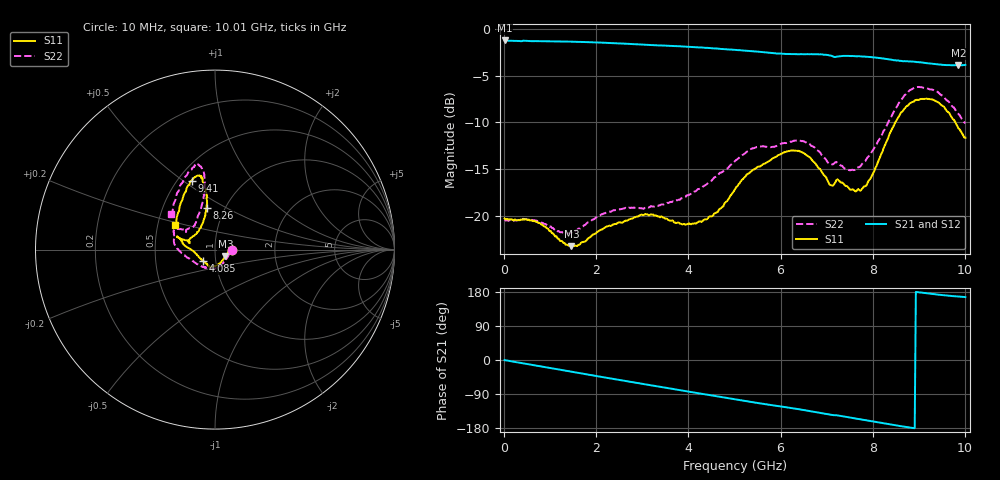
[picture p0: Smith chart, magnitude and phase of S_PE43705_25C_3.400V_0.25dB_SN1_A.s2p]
! Device ID: PE43705
! Serial: 1
! Insertion: A
! Impedance: 50 ohm
! Temp: 25C
! VDD: 3.400V
! Attenuation Step: 0.25dB
#  Hz  S  RI  R  50
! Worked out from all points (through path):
!   401 points, 10 MHz to 10.01 GHz, reference 50 ohm
!   highest |S21| = -1.26 dB at 10 MHz (marker M1); lowest = -3.9 dB at 9.86 GHz (marker M2)
!   group delay of S21, straight-line fit = 55.1 ps
!   lowest |S11| = -23.2 dB at 1.46 GHz (marker M3), VSWR 1.15, Z = 56 - j4.22 ohm
!   |S11| at or under -10 dB: start of sweep to 8.487 GHz; 9.793 GHz to end of sweep
!   |S22| runs from -21.9 to -6.2 dB; largest |S21 - S12| = 0.007
!   S11 on the Smith chart (normalised r, x): 10 MHz: 1.22, -0.00; 4.085 GHz: 0.87, -0.11; 8.26 GHz: 0.82, +0.41; 9.41 GHz: 0.59, +0.54; 10.01 GHz: 0.61, +0.18
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1e7  0.0973 -0.000861  0.8647 -0.0043  0.8654 -0.0041  0.0962 -0.00072
7.1e8  0.0926 0.0127  0.8281 -0.2221  0.8283 -0.2219  0.0945 0.00635
1.46e9  0.0582 -0.0375  0.7313 -0.4365  0.7316 -0.4366  0.0629 -0.0519
1.685e9  0.044 -0.0578  0.6905 -0.4943  0.6905 -0.4944  0.0465 -0.0742
2.235e9  0.00934 -0.0879  0.5704 -0.6155  0.5709 -0.6151  0.00145 -0.1052
3.36e9  -0.0321 -0.0943  0.2749 -0.7658  0.2758 -0.7653  -0.0576 -0.0987
4.085e9  -0.0646 -0.0646  0.0693 -0.7943  0.0698 -0.7942  -0.1131 -0.0723
4.585e9  -0.0986 -0.0321  -0.0717 -0.7811  -0.0709 -0.7807  -0.1557 -0.0444
5.01e9  -0.1392 0.00396  -0.1835 -0.7478  -0.1832 -0.7479  -0.1965 -0.00846
5.41e9  -0.1749 0.0278  -0.2795 -0.7027  -0.2789 -0.7035  -0.2277 0.0356
6.085e9  -0.2078 0.0713  -0.4115 -0.6074  -0.4086 -0.6065  -0.2288 0.0903
6.685e9  -0.1896 0.0594  -0.5227 -0.5099  -0.523 -0.509  -0.2059 0.1162
7.085e9  -0.14 0.0433  -0.5834 -0.4193  -0.5844 -0.4201  -0.1622 0.099
7.26e9  -0.1458 0.0536  -0.5948 -0.3908  -0.5929 -0.3921  -0.1501 0.1162
7.685e9  -0.1001 0.0974  -0.6491 -0.2955  -0.6482 -0.2954  -0.1108 0.145
7.91e9  -0.0754 0.1349  -0.6645 -0.2375  -0.6654 -0.2413  -0.0959 0.1853
8.26e9  -0.0469 0.2336  -0.6744 -0.1501  -0.6717 -0.1553  -0.0645 0.2829
8.36e9  -0.0448 0.2691  -0.6742 -0.1257  -0.6727 -0.1288  -0.0595 0.3208
8.86e9  -0.077 0.3993  -0.6672 -0.00925  -0.6633 -0.0129  -0.0888 0.469
9.41e9  -0.1308 0.3842  -0.6398 0.084  -0.638 0.083  -0.1444 0.4364
9.86e9  -0.1996 0.2154  -0.6212 0.1384  -0.6213 0.1377  -0.2226 0.2714
1.001e10  -0.2229 0.1381  -0.622 0.1552  -0.6243 0.153  -0.2434 0.1974
